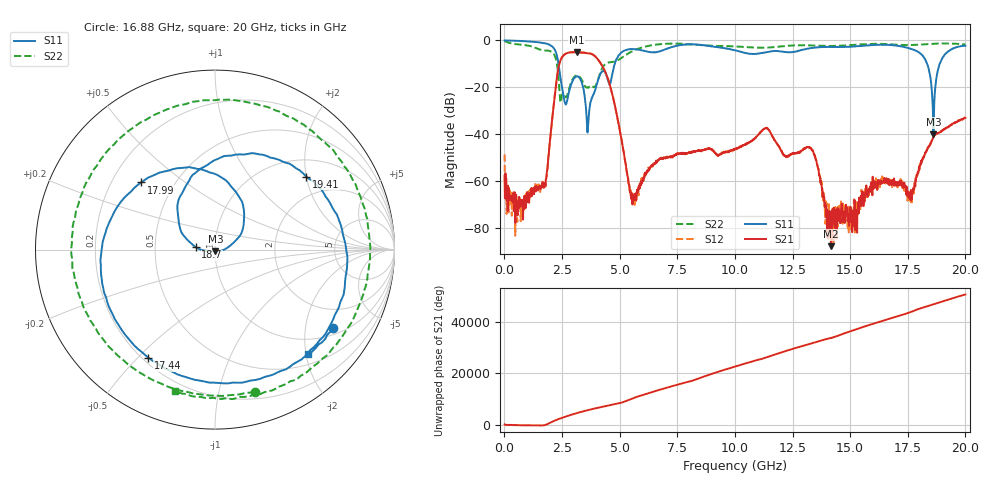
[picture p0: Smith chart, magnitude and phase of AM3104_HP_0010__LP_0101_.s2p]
!Created with skrf (http://scikit-rf.org).
# Hz S RI R 50.0
!freq ReS11 ImS11 ReS21 ImS21 ReS12 ImS12 ReS22 ImS22
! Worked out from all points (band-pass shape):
!   1601 points, 10 MHz to 20 GHz, reference 50 ohm
!   highest |S21| = -4.95 dB at 3.133 GHz (marker M1); lowest = -87.7 dB at 14.17 GHz (marker M2)
!   |S21| within 3 dB of the highest: 2.455 GHz to 4.048 GHz (1.593 GHz wide, 49 % of centre)
!   lowest |S11| = -40.0 dB at 18.61 GHz (marker M3), VSWR 1.02, Z = 50.3 - j0.975 ohm
!   |S11| at or under -10 dB: 2.348 GHz to 4.787 GHz (2.439 GHz wide, 68.4 % of centre); 18.34 GHz to 18.88 GHz (543.4 MHz wide, 2.92 % of centre)
!   |S22| runs from -26.4 to -0.2 dB; largest |S21 - S12| = 0.0056
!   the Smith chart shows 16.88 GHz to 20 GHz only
!   S11 on the Smith chart (normalised r, x): 16.88 GHz: 1.22, -2.85; 17.44 GHz: 0.22, -0.54; 17.99 GHz: 0.32, +0.35; 18.7 GHz: 0.81, +0.02; 19.41 GHz: 1.41, +1.99; 20 GHz: 0.70, -2.03
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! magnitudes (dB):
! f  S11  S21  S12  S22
! 10 MHz  0.0  -57.7  -48.6  -0.2
! 534.7 MHz  -0.1  -69.8  -69.4  -1.6
! 1.697 GHz  -1.1  -61.4  -62.1  -4.2
! 2.384 GHz  -12.4  -10.0  -9.9  -20.5
! 2.659 GHz  -27.3  -5.7  -5.6  -24.2
! 3.133 GHz  -15.3  -4.9  -4.9  -15.0
! 3.346 GHz  -17.5  -5.2  -5.2  -16.6
! 3.621 GHz  -37.7  -5.5  -5.4  -20.0
! 4.47 GHz  -16.1  -15.7  -15.7  -9.5
! 5.532 GHz  -3.7  -66.9  -65.2  -4.7
! 6.682 GHz  -4.8  -51.0  -50.9  -1.7
! 10.01 GHz  -4.2  -46.3  -46.4  -2.5
! 13.34 GHz  -3.2  -46.9  -46.8  -2.1
! 14.17 GHz  -2.8  -87.7  -76.5  -2.3
! 16.68 GHz  -1.9  -60.5  -59.5  -1.6
! 16.88 GHz  -2.0  -60.8  -59.6  -1.7
! 17.44 GHz  -3.0  -65.8  -64.1  -2.0
! 17.99 GHz  -5.1  -53.8  -54.7  -1.8
! 18.61 GHz  -40.0  -41.3  -41.2  -1.4
! 18.7 GHz  -19.4  -40.1  -39.9  -1.4
! 19.41 GHz  -3.7  -35.7  -35.8  -1.3
! 20 GHz  -2.2  -32.9  -32.9  -1.7
